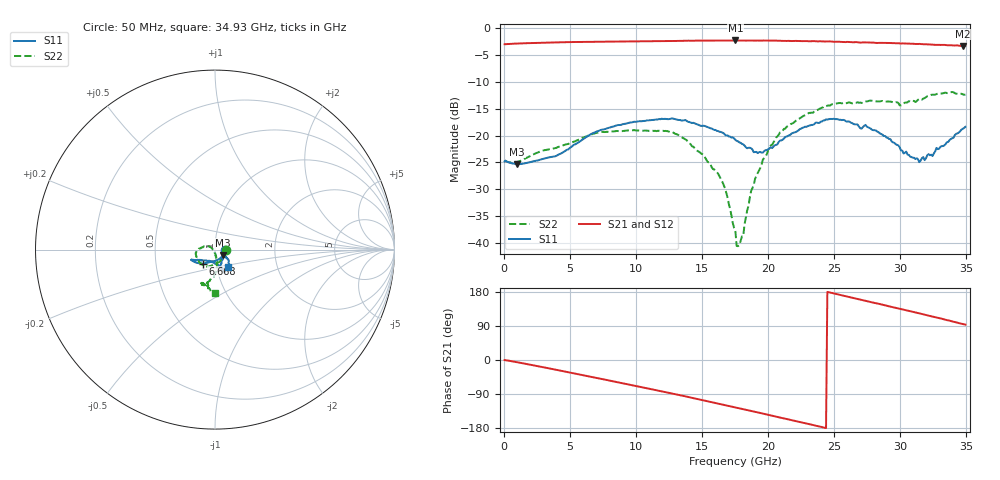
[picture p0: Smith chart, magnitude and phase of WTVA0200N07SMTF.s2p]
! 50 ohm 2-Port S-parameters measured by Modelithics Inc support@modelithics.com  Tampa, FL USA 813-866-6335 (February 2024)
! Smiths Interconnect,  2dB P/N: WTVA0200N07SMTF, Temperature: -50 C
! Board: 10 mil Rogers 4350B, Mounting Pad Dimensions: Length: 15 mils, Width: 25 mils, Gap: 40 mils.
# Hz S RI R 50
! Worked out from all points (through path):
!   352 points, 50 MHz to 34.93 GHz, reference 50 ohm
!   highest |S21| = -2.35 dB at 17.51 GHz (marker M1); lowest = -3.4 dB at 34.73 GHz (marker M2)
!   group delay of S21, straight-line fit = 21.3 ps
!   lowest |S11| = -25.3 dB at 996 MHz (marker M3), VSWR 1.11, Z = 54.5 - j3.42 ohm
!   |S11| at or under -10 dB: start of sweep to end of sweep
!   |S22| runs from -40.6 to -11.9 dB; largest |S21 - S12| = 0.0046
!   S11 on the Smith chart (normalised r, x): 50 MHz: 1.12, -0.01; 6.668 GHz: 0.86, -0.14; 34.93 GHz: 1.13, -0.22
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5e7  0.0575 -0.00255  0.7041 -0.00215  0.7039 -0.00232  0.0589 -0.00251
9.96e8  0.0444 -0.0313  0.7109 -0.0725  0.7107 -0.0725  0.0458 -0.0336
3.8815e9  -0.0057 -0.0639  0.6619 -0.3131  0.6613 -0.3135  0.0124 -0.0753
5.8715e9  -0.0508 -0.0747  0.5721 -0.4683  0.5717 -0.4684  -0.0242 -0.091
6.6675e9  -0.069 -0.0782  0.5252 -0.5231  0.5248 -0.5231  -0.0412 -0.0945
1.1742e10  -0.1287 -0.0605  0.1133 -0.744  0.1122 -0.7439  -0.1053 -0.0342
1.38315e10  -0.124 -0.057  -0.0895 -0.7559  -0.0897 -0.7557  -0.0903 0.00478
1.612e10  -0.0948 -0.0566  -0.3126 -0.6939  -0.3131 -0.6935  -0.0418 0.0185
1.6717e10  -0.0849 -0.057  -0.3677 -0.6668  -0.3683 -0.6663  -0.0289 0.0152
1.7513e10  -0.0692 -0.0595  -0.4392 -0.6243  -0.4396 -0.6237  -0.013 0.00195
1.76125e10  -0.0667 -0.0592  -0.447 -0.6173  -0.4476 -0.6165  -0.00944 8.5e-05
1.811e10  -0.0557 -0.0613  -0.4881 -0.585  -0.4886 -0.5843  -0.00375 -0.011
1.8707e10  -0.0399 -0.0649  -0.5333 -0.5437  -0.5331 -0.5437  0.00325 -0.0304
1.92045e10  -0.0249 -0.064  -0.5691 -0.5063  -0.5693 -0.5058  0.00725 -0.0441
2.01995e10  -0.00136 -0.0779  -0.633 -0.4221  -0.6327 -0.422  0.00824 -0.0808
2.13935e10  0.0248 -0.0944  -0.6879 -0.3108  -0.688 -0.3099  0.00747 -0.1202
2.33835e10  0.0479 -0.116  -0.7438 -0.1119  -0.7436 -0.1113  -0.0219 -0.1612
2.5672e10  0.0566 -0.1278  -0.727 0.1303  -0.7267 0.1304  -0.0643 -0.1907
2.91545e10  0.0288 -0.0883  -0.5664 0.4491  -0.5654 0.4497  -0.0605 -0.1973
3.1443e10  0.0434 -0.0363  -0.3869 0.5945  -0.3858 0.5947  -0.0367 -0.2154
3.47265e10  0.0762 -0.0866  -0.0585 0.6763  -0.0562 0.6762  3.75e-05 -0.2413
3.49255e10  0.0718 -0.0966  -0.0391 0.6782  -0.0359 0.678  -0.00051 -0.2396
